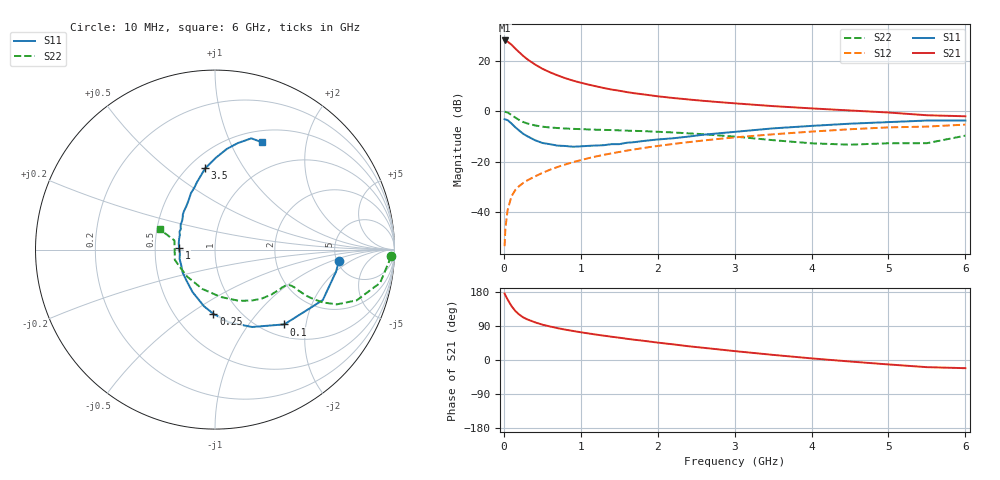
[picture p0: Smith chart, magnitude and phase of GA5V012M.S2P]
! Infineon Technologies  Discrete & RF Semiconductors
! BF775
! Si NPN RF Bipolar Junction Transistor in SOT23
! VCE = 5 V  IC = 12 mA
! Common Emitter S-Parameters:  May  1996
# GHz  S  MA  R  50
!  f  S11  S21  S12  S22
! GHz  MAG  ANG  MAG  ANG  MAG  ANG  MAG  ANG
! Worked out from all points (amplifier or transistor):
!   36 points, 10 MHz to 6 GHz, reference 50 ohm
!   highest |S21| = 28.1 dB at 10 MHz (marker M1)
!   |S21| within 3 dB of that: start of sweep to 141.9 MHz
!   unconditionally stable (mu >= 1): 538.9 MHz to 2.981 GHz
!   at 250 MHz: K = 0.73, MSG = 25.2 dB, |S12| = -28.5 dB
!   at 1.4 GHz: K = 1.10, MAG = 10.7 dB, |S12| = -16.7 dB
!   at 6 GHz: K = 0.93, MSG = 1.7 dB, |S12| = -5.3 dB
!   S11 on the Smith chart (normalised r, x): 10 MHz: 5.21, -1.26; 100 MHz: 1.23, -1.51; 250 MHz: 0.76, -0.62; 1 GHz: 0.67, +0.01; 3.5 GHz: 0.60, +0.69; 6 GHz: 0.63, +1.32
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0.01  0.6933 -5.2  25.29 175.4  0.0021 88.5  0.9832 -2.2
0.02  0.6856 -10.3  24.83 171.0  0.0047 85.3  0.9675 -4.7
0.05  0.6632 -25.1  23.89 159.2  0.0111 79.2  0.9384 -11.4
0.1  0.5679 -47.2  20.81 142.3  0.0206 71.3  0.8384 -19.7
0.15  0.4781 -64.4  17.39 129.1  0.0274 65.2  0.7443 -24.2
0.2  0.4126 -79.2  14.76 119.9  0.0328 64.4  0.6691 -26.1
0.25  0.3574 -91.5  12.55 112.7  0.0375 63.4  0.6117 -26.7
0.3  0.3216 -101.0  10.86 107.6  0.042 63.5  0.5743 -26.8
0.4  0.2675 -117.9  8.535 99.8  0.0504 64.5  0.5235 -26.2
0.5  0.2343 -132.9  6.959 93.3  0.0595 66.0  0.4925 -25.5
0.6  0.2212 -144.6  5.904 88.5  0.069 66.5  0.4751 -25.3
0.7  0.2071 -155.4  5.121 84.0  0.0784 66.9  0.4629 -25.4
0.8  0.204 -165.2  4.509 80.1  0.0877 66.4  0.4527 -25.8
1  0.2006 177.3  3.67 73.2  0.1068 66.4  0.4403 -27.2
1.1  0.2051 170.1  3.369 70.1  0.1169 66.1  0.4347 -28.4
1.3  0.2115 158.0  2.881 64.2  0.1362 64.9  0.4255 -30.6
1.6  0.2368 143.9  2.39 56.0  0.1652 62.5  0.411 -35.0
2.2  0.29 123.4  1.827 41.3  0.2237 57.0  0.3787 -45.8
3.5  0.4561 96.9  1.26 13.5  0.3477 42.0  0.266 -83.0
4.5  0.5647 83.3  1.033 -4.0  0.4382 29.1  0.2165 -136.9
5.5  0.6523 71.9  0.83 -18.9  0.4947 14.2  0.2318 167.3
6  0.6522 66.5  0.792 -21.6  0.5415 10.1  0.3273 159.8
